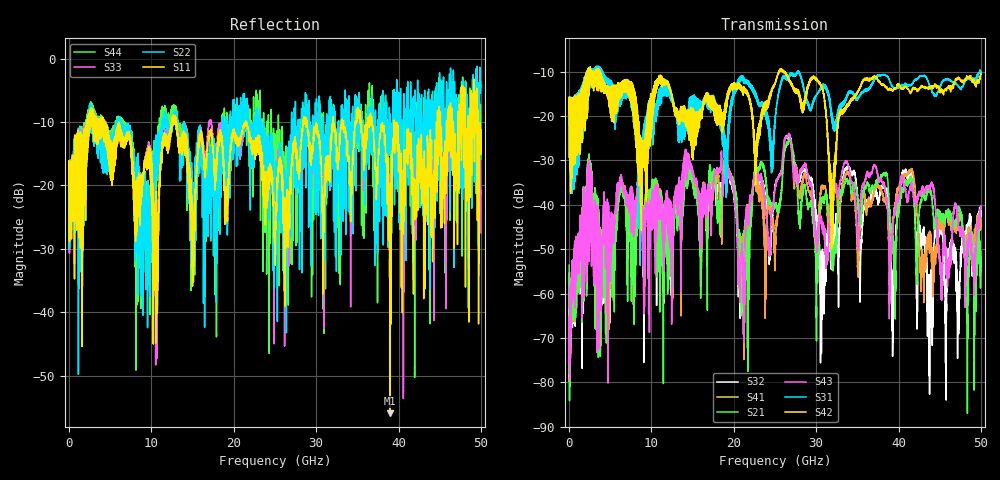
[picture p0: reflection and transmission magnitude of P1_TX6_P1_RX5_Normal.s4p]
!Keysight Technologies,N5225B,MY57041031,A.13.20.10
!Date: Friday, May 31, 2019 11:21:03
!Correction: S11(Full 4 Port(1,2,3,4))
!S12(Full 4 Port(1,2,3,4))
!S13(Full 4 Port(1,2,3,4))
!S14(Full 4 Port(1,2,3,4))
!S21(Full 4 Port(1,2,3,4))
!S22(Full 4 Port(1,2,3,4))
!S23(Full 4 Port(1,2,3,4))
!S24(Full 4 Port(1,2,3,4))
!S31(Full 4 Port(1,2,3,4))
!S32(Full 4 Port(1,2,3,4))
!S33(Full 4 Port(1,2,3,4))
!S34(Full 4 Port(1,2,3,4))
!S41(Full 4 Port(1,2,3,4))
!S42(Full 4 Port(1,2,3,4))
!S43(Full 4 Port(1,2,3,4))
!S44(Full 4 Port(1,2,3,4))
!S4P File: Measurements: <S11,S12,S13,S14>,
!<S21,S22,S23,S24>,
!<S31,S32,S33,S34>,
!<S41,S42,S43,S44>:
# Hz S  dB  R 50.0
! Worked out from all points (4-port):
!   5000 points, 10 MHz to 50 GHz, reference 50 ohm
!   strongest paths, dB at 10 MHz, 12.51 GHz, 25.01 GHz, 37.51 GHz, 50 GHz:
!     S42: -19.5, -15.6, -12.8, -12.1, -10.6
!     S31: -19.4, -15.5, -21.6, -10.8, -9.9
!     S43: -75.9, -55.1, -36.2, -33.5, -40.9
!     S21: -53.6, -47.9, -40.5, -34.7, -54.3
!     S41: -65.0, -48.6, -52.1, -35.6, -43.1
!     S32: -55.4, -51.5, -36.0, -39.6, -40.8
!   lowest |S11| = -56.0 dB at 38.96 GHz (marker M1), VSWR 1.00, Z = 50.1 + j0.069 ohm
!   |S11| at or under -10 dB: 4.286 GHz to 12.47 GHz (8.179 GHz wide, 97.7 % of centre); 13.02 GHz to 21.43 GHz (8.403 GHz wide, 48.8 % of centre); 21.46 GHz to 28.42 GHz (6.96 GHz wide, 27.9 % of centre)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
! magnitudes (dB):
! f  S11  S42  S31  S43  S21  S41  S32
! 10 MHz  -19.4  -19.5  -19.4  -75.9  -53.6  -65.0  -55.4
! 2.45 GHz  -12.1  -11.6  -14.0  -29.7  -28.5  -28.8  -29.2
! 14.32 GHz  -16.7  -19.1  -19.6  -28.5  -30.6  -29.2  -30.1
! 20.99 GHz  -11.4  -14.6  -11.9  -50.2  -59.6  -47.3  -56.4
! 26.57 GHz  -24.8  -11.3  -11.7  -24.5  -26.4  -26.1  -25.1
! 38.96 GHz  -56.0  -13.8  -12.3  -56.9  -41.8  -51.4  -49.1
! 50 GHz  -11.2  -10.6  -9.9  -40.9  -54.3  -43.1  -40.8
